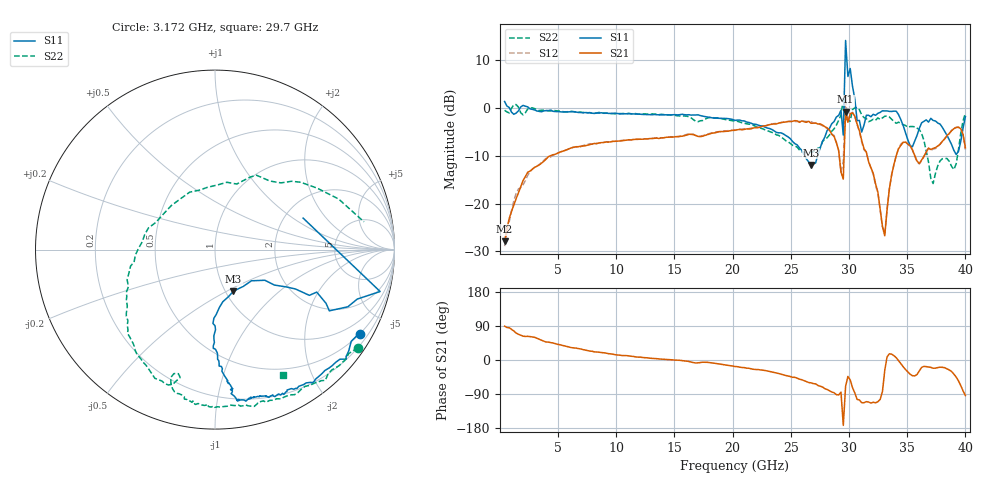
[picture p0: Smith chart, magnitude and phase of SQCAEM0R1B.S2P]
! Network Analyzer HP8722ES.07.66: Jul 25, 2000 Serial No. US39175408
! 26 Oct 2004  08:24:39
! Frequency  S11  S21  S12  S22
# HZ  S  DB R  50
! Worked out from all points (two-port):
!   201 points, 400 MHz to 40 GHz, reference 50 ohm
!   highest |S21| = -0.76 dB at 29.7 GHz (marker M1); lowest = -27.9 dB at 400 MHz (marker M2)
!   |S21| within 3 dB of the highest: 22.64 GHz to 27.84 GHz (5.202 GHz wide, 20.6 % of centre); 29.66 GHz to 30.75 GHz (1.091 GHz wide, 3.61 % of centre)
!   lowest |S11| = -11.9 dB at 26.73 GHz (marker M3), VSWR 1.68, Z = 54.5 - j27 ohm
!   |S11| at or under -10 dB: 26.19 GHz to 27.3 GHz (1.104 GHz wide, 4.13 % of centre)
!   |S22| runs from -15.8 to 2.0 dB; largest |S21 - S12| = 0.52
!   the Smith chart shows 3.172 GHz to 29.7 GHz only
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4e8  1.39 -0.3  -27.91 89.3  -28.90 92.9  -0.46 5.0
2.578e9  -0.15 -25.6  -13.18 61.8  -13.38 59.3  0.02 -32.1
7.132e9  -0.98 -58.5  -7.94 27.5  -7.85 26.4  -0.93 -67.6
1.3666e10  -1.40 -75.4  -6.36 2.8  -6.23 2.9  -1.39 -98.3
2.02e10  -2.56 -84.3  -4.65 -17.2  -4.54 -16.5  -2.72 -125.3
2.6734e10  -11.93 -66.1  -3.18 -60.4  -2.85 -60.0  -9.30 105.1
2.6932e10  -11.75 -52.4  -3.15 -62.3  -3.07 -61.3  -9.12 96.6
2.9308e10  -0.45 -14.2  -13.43 -84.7  -13.34 -83.2  -1.47 10.6
2.9506e10  -5.66 19.7  -14.87 -172.6  -11.12 -138.4  1.99 28.1
2.9704e10  14.16 -50.0  -0.76 -69.5  1.81 -47.4  -2.01 -61.4
2.9902e10  6.62 -58.2  -2.98 -43.4  -3.02 -42.6  -2.66 3.0
3.01e10  8.29 -75.8  -1.21 -52.3  -1.18 -51.6  -2.72 3.3
3.0496e10  1.93 -85.7  -1.71 -86.9  -1.69 -85.3  0.05 -30.1
3.0694e10  -2.62 96.3  -3.35 -104.0  -3.42 -102.5  0.12 135.3
3.1288e10  -3.56 136.0  -8.51 -112.7  -8.74 -113.0  -1.98 121.7
3.1486e10  -1.52 -43.7  -9.19 -109.9  -9.23 -110.7  -2.18 -60.2
3.307e10  -0.60 -47.6  -26.72 -27.5  -26.29 -24.9  -1.71 -80.1
3.3466e10  -0.69 -53.6  -16.91 16.4  -16.90 18.0  -1.87 -82.1
3.5644e10  -6.91 -45.3  -9.92 -42.0  -10.08 -41.1  -3.91 -93.4
3.7228e10  -2.59 -73.3  -8.44 -21.6  -8.54 -20.2  -15.79 -65.2
3.901e10  -8.84 -78.0  -4.31 -37.2  -4.23 -36.9  -12.87 -18.4
4e10  -1.78 -35.0  -8.31 -93.7  -8.69 -93.0  -1.07 -8.5
